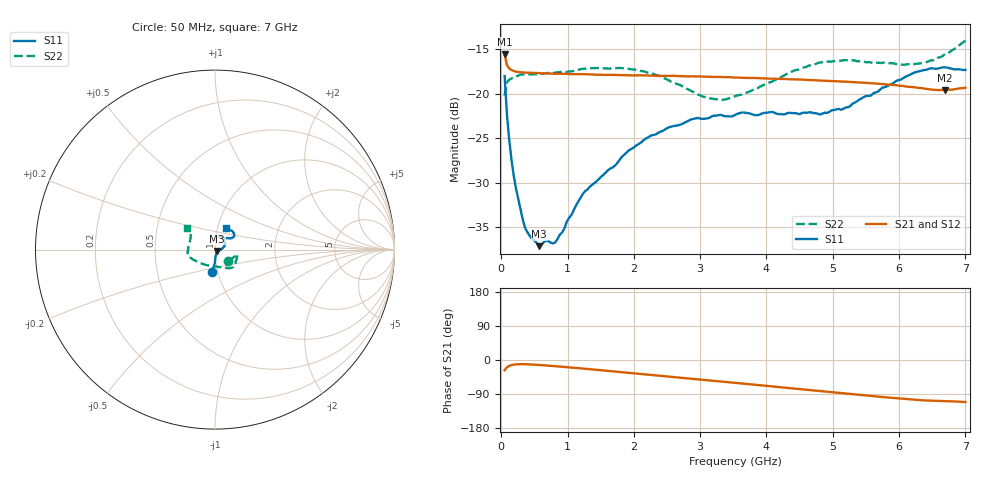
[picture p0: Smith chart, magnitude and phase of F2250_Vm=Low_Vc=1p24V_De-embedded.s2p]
! Integrated Device Technology
! Corporate Headquarters
! 6024 Silver Creek Valley Road
! San Jose, CA 95138  USA
! Phone:  1-408-284-8200
! Toll Free:  1-800-223-1366
! Webpage:  http://www.idt.com/
! Timing and RF Division
! 515 Groton Road, Suite 102
! Westford, MA 01886-6024
! Device:  F2250
! Description: Voltage Variable RF Attenuator
! Frequency:  50.0 -  6000.00 MHz
! Package:  3x3 mm Thin QFN Plastic Package: 16 pin
! Ports:  2 RF, 3 DC
!  Pin  1  = GND
!  Pin  2  = NC
!  Pin  3  = RF1  = Port 1
!  Pin  4  = NC
!  Pin  5  = GND
!  Pin  6  = GND
!  Pin  7  = GND
!  Pin  8  = GND
!  Pin  9  = NC
!  Pin 10  = RF2  = Port 2
!  Pin 11  = NC
!  Pin 12  = GND
!  Pin 13  = GND
!  Pin 14  = VCNTRL
!  Pin 15  = VDD
!  Pin 16  = VMODE
! Vcntrl:  1.240 Volts
! Vmode:  +0.000 Volts
! Vdd:  +3.30  Volts
! Current:  1.192 mA
! Data:  The device was measured on a the F2250 evaluation board which has
!  individual transmission lines to the RF pins.  Data was collected
!  using a calibrated network analyzer.  The evaluation board was
!  de-embedded using a TRL calibration technique.
!  The reference plane is the edge of the package pin.
! Misc:  SN 10
!  Action Tracker AT0258
! Date Measured:  2014-11-26
! Date:  2015-10-15  MJV
! Note:
!  Integrated Device Technology supplies this data as a sample of measured
!  data at the package pin for this product.  Your particular data for this
!  product may vary.
!  Data was taken at 25 degrees C.
!  Integrated Device Technology reserves the right to change this data at anytime.
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# GHz S dB R 50
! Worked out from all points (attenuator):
!   201 points, 50 MHz to 7 GHz, reference 50 ohm
!   highest |S21| = -15.57 dB at 50 MHz (marker M1); lowest = -19.6 dB at 6.687 GHz (marker M2)
!   lowest |S11| = -37.2 dB at 571.2 MHz (marker M3), VSWR 1.03, Z = 51.1 - j0.845 ohm
!   |S11| at or under -10 dB: start of sweep to end of sweep
!   |S22| runs from -20.7 to -14.0 dB; largest |S21 - S12| = 0.00068
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0.05  -17.99 -98.2  -15.57 -27.1  -15.54 -27.1  -20.23 -40.0
0.08475  -22.29 -90.8  -16.74 -19.4  -16.72 -19.4  -18.70 -19.3
0.1195  -25.20 -88.8  -17.14 -15.5  -17.12 -15.5  -18.41 -14.0
0.189  -29.32 -83.2  -17.43 -12.2  -17.44 -12.2  -18.12 -11.9
0.22375  -30.75 -78.5  -17.51 -11.5  -17.49 -11.5  -18.04 -12.3
0.36275  -35.20 -64.2  -17.61 -11.2  -17.59 -11.2  -17.83 -13.2
0.57125  -37.18 -36.7  -17.66 -13.1  -17.68 -13.1  -17.78 -18.2
0.6755  -36.57 -32.4  -17.70 -14.4  -17.69 -14.4  -17.67 -20.9
0.8145  -36.74 -20.1  -17.74 -16.3  -17.72 -16.3  -17.61 -24.8
1.2315  -31.27 -6.6  -17.79 -22.6  -17.78 -22.6  -17.18 -34.6
1.9265  -26.36 14.4  -17.91 -33.7  -17.90 -33.7  -17.19 -46.3
2.37825  -24.35 25.9  -17.98 -41.0  -17.97 -41.0  -17.95 -55.1
2.86475  -22.88 41.1  -18.02 -49.2  -18.01 -49.2  -19.67 -72.3
3.07325  -22.80 47.9  -18.06 -52.7  -18.07 -52.7  -20.38 -83.7
3.3165  -22.38 56.3  -18.10 -56.8  -18.09 -56.8  -20.68 -100.3
3.525  -22.38 61.2  -18.17 -60.2  -18.17 -60.3  -20.27 -114.5
4.7065  -22.18 67.0  -18.45 -80.2  -18.46 -80.2  -16.72 -162.5
5.22775  -21.51 49.9  -18.64 -89.0  -18.67 -89.0  -16.21 -172.1
5.85325  -19.00 35.0  -18.96 -99.3  -18.97 -99.4  -16.55 174.0
6.33975  -17.39 37.4  -19.35 -106.2  -19.38 -106.2  -16.54 156.8
6.68725  -17.00 46.4  -19.58 -108.6  -19.58 -108.6  -15.55 144.7
7  -17.31 63.0  -19.31 -110.8  -19.27 -111.0  -13.98 142.6
